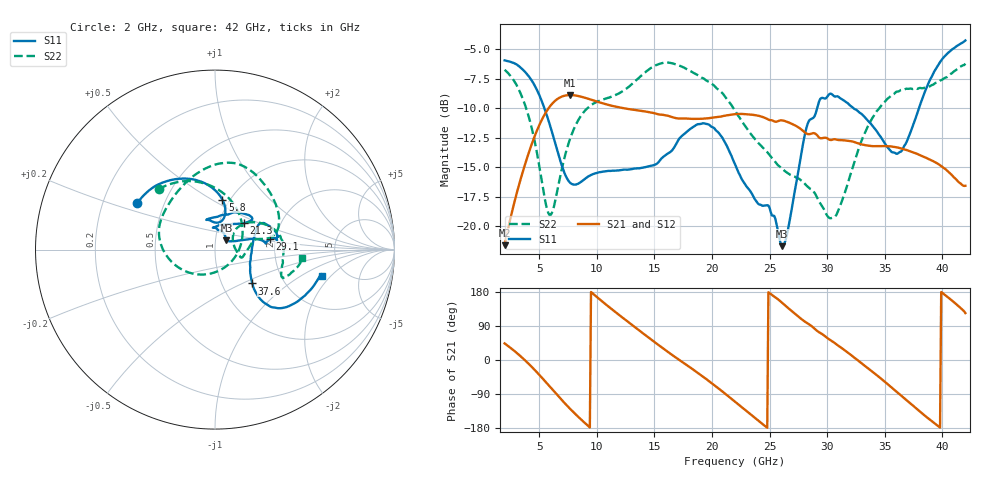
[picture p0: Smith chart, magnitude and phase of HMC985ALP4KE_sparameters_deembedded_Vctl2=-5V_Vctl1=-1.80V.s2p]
!s2p File: Measurements: S11, S21, S12, S22
# GHz S dB R 50.0
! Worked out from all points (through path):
!   401 points, 2 GHz to 42 GHz, reference 50 ohm
!   highest |S21| = -8.88 dB at 7.7 GHz (marker M1); lowest = -21.6 dB at 2 GHz (marker M2)
!   lowest |S11| = -21.7 dB at 26.1 GHz (marker M3), VSWR 1.18, Z = 56.4 + j5.98 ohm
!   |S11| at or under -10 dB: 5.454 GHz to 29.13 GHz (23.67 GHz wide, 137 % of centre); 32.29 GHz to 37.97 GHz (5.675 GHz wide, 16.2 % of centre)
!   |S22| runs from -19.3 to -6.1 dB; largest |S21 - S12| = 0.00039
!   S11 on the Smith chart (normalised r, x): 2 GHz: 0.35, +0.24; 5.8 GHz: 0.92, +0.56; 21.3 GHz: 1.31, +0.41; 29.1 GHz: 1.86, +0.24; 37.6 GHz: 1.39, -0.57; 42 GHz: 3.36, -1.58
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2  -5.94 149.1  -21.60 43.8  -21.61 43.8  -6.74 133.1
3.2  -6.40 129.9  -16.66 14.9  -16.67 14.9  -8.35 102.1
4.4  -7.71 107.7  -12.91 -19.5  -12.92 -19.5  -11.86 61.3
5.8  -11.00 81.6  -10.02 -65.9  -10.02 -65.9  -18.89 -33.9
7.7  -16.32 82.0  -8.88 -129.3  -8.88 -129.3  -12.54 -158.1
8.7  -16.19 94.4  -9.03 -158.8  -9.04 -158.8  -10.54 176.8
10.2  -15.42 102.6  -9.49 161.4  -9.49 161.4  -9.38 154.5
12.2  -15.22 106.1  -9.97 112.7  -9.97 112.7  -8.58 129.0
15.4  -14.52 83.3  -10.52 38.7  -10.52 38.7  -6.25 83.2
18.2  -11.69 49.6  -10.89 -21.6  -10.90 -21.6  -6.88 51.3
21.3  -13.20 42.5  -10.60 -92.7  -10.60 -92.7  -9.22 14.7
22  -14.73 51.3  -10.50 -110.1  -10.51 -110.1  -10.20 12.1
24.1  -18.15 92.2  -10.65 -161.7  -10.65 -161.7  -13.02 13.5
26.1  -21.68 39.7  -11.03 150.6  -11.03 150.6  -15.13 -3.3
28.7  -10.86 6.7  -12.12 88.1  -12.13 88.2  -16.90 -14.6
29.1  -10.11 10.9  -12.25 77.5  -12.26 77.5  -17.51 -12.2
30.7  -9.01 13.9  -12.62 43.7  -12.63 43.7  -19.16 24.9
32.9  -10.42 29.3  -13.04 -6.4  -13.04 -6.4  -12.97 40.8
35.4  -13.47 7.5  -13.22 -67.6  -13.23 -67.6  -9.07 17.6
37.6  -11.05 -42.2  -13.79 -124.6  -13.79 -124.6  -8.31 -5.8
39.8  -6.09 -41.0  -14.83 -178.3  -14.82 -178.3  -7.66 -22.4
42  -4.26 -13.9  -16.56 123.7  -16.57 123.7  -6.22 -5.3
